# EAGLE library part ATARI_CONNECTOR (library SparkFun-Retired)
DB9 labeled for Atari joystick
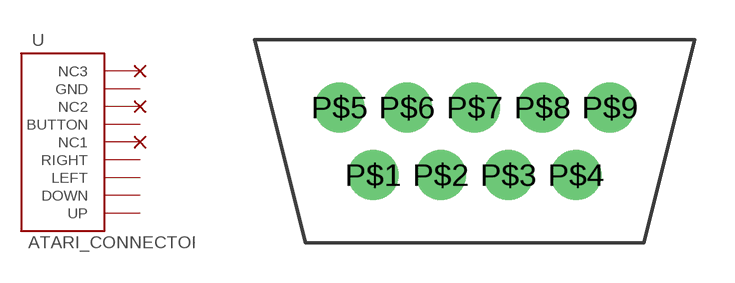
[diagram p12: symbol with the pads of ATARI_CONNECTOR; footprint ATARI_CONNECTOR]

Designator prefix -

## ATARI_CONNECTOR  [ATARI_CONNECTOR]
P$1  BUTTON
P$2  NC2
P$3  GND
P$4  NC3
P$5  UP
P$6  DOWN
P$7  LEFT
P$8  RIGHT
P$9  NC1

## Footprint ATARI_CONNECTOR (pad centres in mm)
drill 0.8 pad 1.88: P$1 1.27,2.54; P$2 3.81,2.54; P$3 6.35,2.54; P$4 8.89,2.54; P$5 0,5.08; P$6 2.54,5.08; P$7 5.08,5.08; P$8 7.62,5.08; P$9 10.16,5.08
